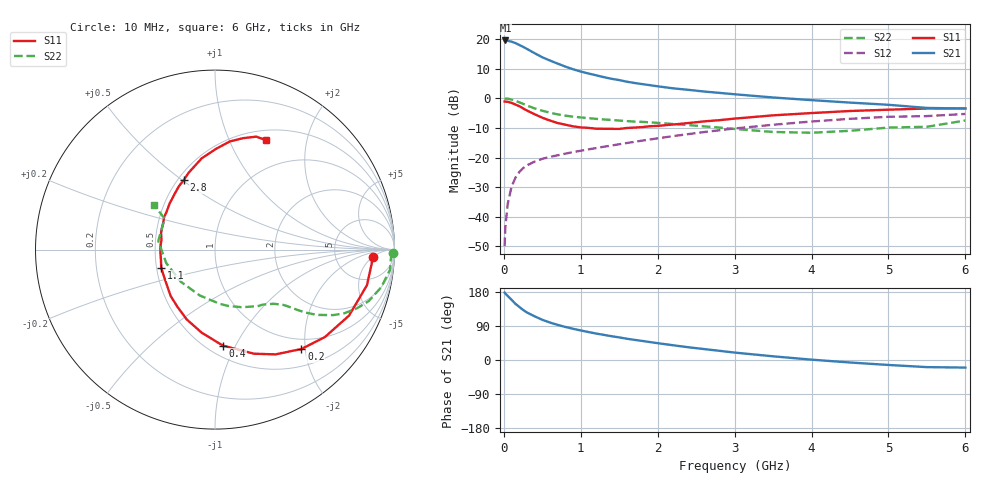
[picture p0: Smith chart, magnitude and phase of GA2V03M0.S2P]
! Infineon Technologies  Discrete & RF Semiconductors
! BF775
! Si NPN RF Bipolar Junction Transistor in SOT23
! VCE = 2 V  IC = 3 mA
! Common Emitter S-Parameters:  May  1996
# GHz  S  MA  R  50
!  f  S11  S21  S12  S22
! GHz  MAG  ANG  MAG  ANG  MAG  ANG  MAG  ANG
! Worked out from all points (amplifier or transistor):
!   36 points, 10 MHz to 6 GHz, reference 50 ohm
!   highest |S21| = 19.5 dB at 20 MHz (marker M1)
!   |S21| within 3 dB of that: start of sweep to 310.8 MHz
!   unconditionally stable (mu >= 1): 958.6 MHz to 4.139 GHz; 5.163 GHz to end of sweep
!   at 250 MHz: K = 0.37, MSG = 20.5 dB, |S12| = -23.6 dB
!   at 1.4 GHz: K = 1.14, MAG = 9.0 dB, |S12| = -16.0 dB
!   at 6 GHz: K = 1.00, MAG = 0.5 dB, |S12| = -5.3 dB
!   S11 on the Smith chart (normalised r, x): 10 MHz: 14, -5; 200 MHz: 0.80, -1.92; 400 MHz: 0.59, -0.89; 1.1 GHz: 0.53, -0.12; 2.8 GHz: 0.54, +0.51; 6 GHz: 0.62, +1.38
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0.01  0.8789 -2.7  9.343 178.0  0.0032 90.3  0.9946 -1.2
0.02  0.8763 -5.3  9.406 175.4  0.0068 88.4  0.9812 -2.7
0.05  0.8696 -13.2  9.276 169.2  0.0164 83.1  0.9816 -6.6
0.1  0.8325 -26.2  8.975 159.0  0.0322 75.0  0.9496 -12.8
0.15  0.7826 -38.5  8.497 148.4  0.0454 68.7  0.9033 -18.5
0.2  0.734 -49.0  7.904 140.2  0.0568 64.1  0.8543 -22.6
0.25  0.674 -60.0  7.35 132.2  0.0661 59.7  0.8033 -26.2
0.3  0.6193 -69.5  6.78 125.4  0.0736 56.6  0.7531 -29.0
0.4  0.5368 -85.3  5.738 115.3  0.0853 52.2  0.6734 -32.7
0.5  0.4688 -99.1  4.896 106.1  0.0951 49.7  0.6149 -34.8
0.6  0.4196 -112.1  4.311 98.8  0.1024 48.5  0.5687 -36.2
0.7  0.3808 -123.5  3.826 92.6  0.1091 48.0  0.5338 -37.3
0.9  0.3355 -142.3  3.074 82.4  0.1235 47.6  0.4884 -39.1
1.1  0.3161 -161.4  2.61 73.8  0.1372 48.1  0.4607 -41.3
1.3  0.3048 -176.7  2.263 66.3  0.152 48.7  0.438 -43.6
1.6  0.3146 162.7  1.896 56.1  0.1756 49.0  0.4107 -48.1
2.2  0.3604 134.6  1.466 38.9  0.2294 47.4  0.3677 -60.2
2.8  0.4259 113.9  1.23 24.3  0.2878 43.1  0.32 -77.8
3.5  0.5138 98.3  1.028 9.7  0.3566 35.7  0.2695 -108.1
4.5  0.6081 82.2  0.843 -6.6  0.449 23.0  0.282 -164.7
5.5  0.6701 69.9  0.685 -18.8  0.4988 8.0  0.3294 148.5
6  0.6726 64.8  0.669 -20.0  0.5427 3.9  0.421 143.7
